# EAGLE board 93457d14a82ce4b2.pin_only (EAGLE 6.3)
REV: D

Size 66.04 x 50.8 mm. Coordinates in mm from the lower left corner, seen from the top.
Outline: 0,45.72 0,5.08 arc90 5.08,0 60.96,0 arc90 66.04,5.08 66.04,45.72 arc90 60.96,50.8 5.08,50.8 arc90 0,45.72
Copper layers (1*16): Top 0.035mm / dielectric 1.5mm / Bottom 0.035mm
Design rules "adafruit": minimum track width 8mil, minimum drill 15.5mil, track to track 8mil, track to pad 8mil, pad to pad 8mil, via to via 8mil, smd to smd 8mil, copper to edge 10mil, drill to drill 8mil, minimum pad ring 10mil, minimum via ring 8mil, stop-mask expansion 2mil, vias tented up to drill 20mil, thermal gap 10mil
tRestrict: area 24.7,24.1 to 24.8,24.4; area 7,19.9 to 7.5,20; area 22.1,34.8 to 22.9,36.2; area 22.2,32.8 to 22.9,34.2; area 22.2,31.8 to 22.7,32.3; area 22.2,30.2 to 22.9,31.1; area 22.4,27.3 to 22.7,29.7; area 23.2,25.3 to 24.3,25.9; area 25.3,25.3 to 31.1,25.8; area 49.5,9.7 to 49.9,9.8; 1 lines

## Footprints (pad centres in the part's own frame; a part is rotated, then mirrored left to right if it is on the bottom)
0805-NO = smd 1.3 x 1.5: 1 -0.95,0; 2 0.95,0
_0805MP = smd 1.2 x 1.3: 1 -1.016,0; 2 1.016,0
PANASONIC_C = smd 2.6 x 1.4: + 2.05,0; - -2.05,0
SOD-123 = smd 1.4 x 1.4: A 1.85,0; C -1.85,0
SMADIODE = smd 2.54 x 2.54: A 2.349,0; C -2.349,0
SOD-323 = smd 1.35 x 0.8: A 1.27,0; C -1.27,0
FIDUCIAL_1MM = smd 1 x 1: 1 0,0
TSSOP20-5.3MMBODY = smd 0.305 x 1.27: 1 -2.925,-3.618; 2 -2.275,-3.618; 3 -1.625,-3.618; 4 -0.975,-3.618; 5 -0.325,-3.618; 6 0.325,-3.618; 7 0.975,-3.618; 8 1.625,-3.618; 9 2.275,-3.618; 10 2.925,-3.618; 11 2.925,3.618; 12 2.275,3.618; 13 1.625,3.618; 14 0.975,3.618; 15 0.325,3.618; 16 -0.325,3.618; 17 -0.975,3.618; 18 -1.625,3.618; 19 -2.275,3.618; 20 -2.925,3.618
1X02_ROUND = drill 1 pad 1.778: 1 -1.27,0; 2 1.27,0
1X04_ROUND_76 = drill 1 pad 1.93: 1 -3.81,0; 2 -1.27,0; 3 1.27,0; 4 3.81,0
INDUCTOR_5X5MM_NR5040_NOTHERMALS = smd 1.8 x 4: P$1 -1.8,0; P$2 1.8,0
CHIPLED_0805_NOOUTLINE = smd 1.2 x 1.2: A 0,-1.05; C 0,1.05
SOT23-R = smd 0.635 x 1.016: 1 -0.95,-1; 2 0.95,-1; 3 0,1
RESPACK_4X0603 = smd 0.45 x 0.9: 1 -1.3,-0.85; 2 -0.4,-0.85; 3 0.4,-0.85; 4 1.3,-0.85; 5 1.3,0.85; 6 0.4,0.85; 7 -0.4,0.85; 8 -1.3,0.85
SOLDERJUMPER_ARROW_NOPASTE = smd 0.762 x 1.524: 1 -1.016,0; 2 1.016,0
SOLDERJUMPER_CLOSEDWIRE = smd 1.168 x 1.6: 1 -0.762,0; 2 0.762,0 | smd 0.635 x 0.203: WIRE 0,0
S-PQFP-G100 = smd 0.27 x 1.5: 1 -6,-7.75; 2 -5.5,-7.75; 3 -5,-7.75; 4 -4.5,-7.75; 5 -4,-7.75; 6 -3.5,-7.75; 7 -3,-7.75; 8 -2.5,-7.75; 9 -2,-7.75; 10 -1.5,-7.75; 11 -1,-7.75; 12 -0.5,-7.75; 13 0,-7.75; 14 0.5,-7.75; 15 1,-7.75; 16 1.5,-7.75; 17 2,-7.75; 18 2.5,-7.75; 19 3,-7.75; 20 3.5,-7.75; 21 4,-7.75; 22 4.5,-7.75; 23 5,-7.75; 24 5.5,-7.75; 25 6,-7.75; 51 6,7.75; 52 5.5,7.75; 53 5,7.75; 54 4.5,7.75; 55 4,7.75; 56 3.5,7.75; 57 3,7.75; 58 2.5,7.75; 59 2,7.75; 60 1.5,7.75; 61 1,7.75; 62 0.5,7.75; 63 0,7.75; 64 -0.5,7.75; 65 -1,7.75; 66 -1.5,7.75; 67 -2,7.75; 68 -2.5,7.75; 69 -3,7.75; 70 -3.5,7.75; 71 -4,7.75; 72 -4.5,7.75; 73 -5,7.75; 74 -5.5,7.75; 75 -6,7.75 | smd 1.5 x 0.27: 26 7.75,-6; 27 7.75,-5.5; 28 7.75,-5; 29 7.75,-4.5; 30 7.75,-4; 31 7.75,-3.5; 32 7.75,-3; 33 7.75,-2.5; 34 7.75,-2; 35 7.75,-1.5; 36 7.75,-1; 37 7.75,-0.5; 38 7.75,0; 39 7.75,0.5; 40 7.75,1; 41 7.75,1.5; 42 7.75,2; 43 7.75,2.5; 44 7.75,3; 45 7.75,3.5; 46 7.75,4; 47 7.75,4.5; 48 7.75,5; 49 7.75,5.5; 50 7.75,6; 76 -7.75,6; 77 -7.75,5.5; 78 -7.75,5; 79 -7.75,4.5; 80 -7.75,4; 81 -7.75,3.5; 82 -7.75,3; 83 -7.75,2.5; 84 -7.75,2; 85 -7.75,1.5; 86 -7.75,1; 87 -7.75,0.5; 88 -7.75,0; 89 -7.75,-0.5; 90 -7.75,-1; 91 -7.75,-1.5; 92 -7.75,-2; 93 -7.75,-2.5; 94 -7.75,-3; 95 -7.75,-3.5; 96 -7.75,-4; 97 -7.75,-4.5; 98 -7.75,-5; 99 -7.75,-5.5; 100 -7.75,-6 | drill 0.4: P$1 -4,4; P$2 -2,4; P$3 0,4; P$4 2,4; P$5 4,4; P$6 4,2; P$7 4,0; P$8 4,-2; P$9 4,-4; P$10 2,-4; P$11 0,-4; P$12 -2,-4; P$13 -4,-4; P$14 -4,-2; P$15 -4,0; P$16 -4,2 | smd 12 x 12: THERMAL 0,0
SOT23-5 = smd 0.55 x 1.2: 1 -0.95,-1.3; 2 0,-1.3; 3 0.95,-1.3; 4 0.95,1.3; 5 -0.95,1.3
SOT223-R = smd 1.3 x 1.3: 1 -2.3,-3.05; 2 0,-3.05; 3 2.3,-3.05 | smd 3.6 x 1.3: 4 0,3.05
MOUNTINGHOLE_3.0_PLATED = drill 3 pad 6.452: P$1 0,0
HDMI_MOLEX_47151-0001_DIMLAYER = smd 0.25 x 2.6: 1 4.5,0; 2 4,0; 3 3.5,0; 4 3,0; 5 2.5,0; 6 2,0; 7 1.5,0; 8 1,0; 9 0.5,0; 10 0,0; 11 -0.5,0; 12 -1,0; 13 -1.5,0; 14 -2,0; 15 -2.5,0; 16 -3,0; 17 -3.5,0; 18 -4,0; 19 -4.5,0 | drill 0.9 pad 1.65 long: P$1 -7.25,-0.76; P$2 7.25,-0.76 | drill 0.9 pad 1.5 long: P$3 7.25,-6.72; P$4 -7.25,-6.72
4UCONN_20329 = smd 1 x 2: BASE@1 -0.75,-2; BASE@2 0.75,-2 | smd 0.4 x 1.35: D+ 0,0.775; D- -0.65,0.775; GND 1.3,0.775; ID 0.65,0.775; VBUS -1.3,0.775 | drill 0.7 offset: SPRT@1 -3.3,0.9; SPRT@2 3.3,0.9 | drill 0.6 pad 2.5 square: SPRT@3 -3.6,-1.9; SPRT@4 3.6,-1.9 | hole 0.7: -1.95,0; 1.95,0
4-1734839-0 = smd 0.25 x 1.1: 1 -9.75,-2.54; 2 -9.25,-2.54; 3 -8.75,-2.54; 4 -8.25,-2.54; 5 -7.75,-2.54; 6 -7.25,-2.54; 7 -6.75,-2.54; 8 -6.25,-2.54; 9 -5.75,-2.54; 10 -5.25,-2.54; 11 -4.75,-2.54; 12 -4.25,-2.54; 13 -3.75,-2.54; 14 -3.25,-2.54; 15 -2.75,-2.54; 16 -2.25,-2.54; 17 -1.75,-2.54; 18 -1.25,-2.54; 19 -0.75,-2.54; 20 -0.25,-2.54; 21 0.25,-2.54; 22 0.75,-2.54; 23 1.25,-2.54; 24 1.75,-2.54; 25 2.25,-2.54; 26 2.75,-2.54; 27 3.25,-2.54; 28 3.75,-2.54; 29 4.25,-2.54; 30 4.75,-2.54; 31 5.25,-2.54; 32 5.75,-2.54; 33 6.25,-2.54; 34 6.75,-2.54; 35 7.25,-2.54; 36 7.75,-2.54; 37 8.25,-2.54; 38 8.75,-2.54; 39 9.25,-2.54; 40 9.75,-2.54 | smd 2.3 x 3.1: M1 11.4,-0.84; M2 -11.4,-0.84
RESONATOR-SMD = smd 0.7 x 1.7: 1 -1.2,0; 2 0,0; 3 1.2,0

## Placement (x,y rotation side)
C1  0.1uF  [0805-NO]  48.39,3.56 0 top
C2  0.1uF  [0805-NO]  26.3,20 270 top
C3  0.1uF  [0805-NO]  27.05,41.8 180 top
C4  0.1uF  [0805-NO]  43.56,3.3 0 top
C5  0.1uF  [0805-NO]  41.2,26.87 0 top
C6  0.1uF  [_0805MP]  40.8,35 90 top
C7  0.1uF  [0805-NO]  31.75,41.8 180 top
C8  0.1uF  [0805-NO]  20.25,40.25 0 top
C9  0.1uF  [0805-NO]  14.7,15.55 270 top
C10  0.1uF  [0805-NO]  20,20 270 top
C11  0.1uF  [0805-NO]  14.5,27.25 270 top
C12  10uF  [0805-NO]  12.42,14.41 270 top
C13  10uF  [0805-NO]  13.9,7.3 90 top
C14  10uF  [0805-NO]  22.9,7.3 90 top
C15  10uF  [0805-NO]  41.2,23.4 180 top
C16  10uF  [0805-NO]  37.52,45.33 270 top
C17  1uF  [0805-NO]  54,42.5 90 top
C18  1uF  [0805-NO]  51.8,42.5 90 top
C19  0.1uF  [0805-NO]  45,47.1 270 top
C20  0.1uF  [0805-NO]  24.3,42.9 270 top
C21  0.01uF  [0805-NO]  55.37,9.27 270 top
C22  0.01uF  [0805-NO]  59.31,10.29 180 top
C23  0.1uF  [0805-NO]  26.67,6.22 90 top
C24  0.01uF  [0805-NO]  53.98,12.7 270 top
C25  0.01uF  [0805-NO]  52.2,11.05 270 top
C26  100uF  [PANASONIC_C]  9.78,19.05 180 top
D1  MBR0540  [SOD-123]  47.3,40.2 180 top
D2  MM3Z24VT1G  [SMADIODE]  48.8,45.1 90 top
D3  2N4148  [SOD-323]  53.09,47.24 90 top
FB1  Ferrite  [_0805MP]  20.2,15.55 90 top
FB2  Ferrite  [_0805MP]  41.2,25.2 180 top
FB3  Ferrite  [_0805MP]  16.6,15.55 90 top
FB4  Ferrite  [_0805MP]  18.4,15.55 90 top
FB5  ferrite  [_0805MP]  57.66,12.06 0 top
FB6  ferrite  [_0805MP]  62.99,10.29 0 top
FB7  Ferrite  [_0805MP]  48.39,1.91 180 top
FB8  Ferrite  [_0805MP]  37.97,7.49 0 top
FB9  ferrite  [_0805MP]  56.52,16.38 0 top
FB10  ferrite  [_0805MP]  56.64,14.61 0 top
FID1  FIDUCIAL""  [FIDUCIAL_1MM]  37.19,41.95 0 top
FID2  FIDUCIAL""  [FIDUCIAL_1MM]  8.26,9.51 0 top
FID3  FIDUCIAL""  [FIDUCIAL_1MM]  45.88,14.76 0 top
IC1  AR1100_SSOP  [TSSOP20-5.3MMBODY]  46.1,7.75 90 top
JP1  [1X02_ROUND]  64.77,39.37 270 top
JP2  [1X02_ROUND]  2.92,21.34 0 top
JP6  [1X02_ROUND]  11.6,2.2 180 top
JP7  [1X04_ROUND_76]  13.97,48.26 0 top
L1  BRL3225T150K  [INDUCTOR_5X5MM_NR5040_NOTHERMALS]  41.5,41.4 0 top
LED1  Red  [CHIPLED_0805_NOOUTLINE]  54.48,2.04 270 top
LED2  Green  [CHIPLED_0805_NOOUTLINE]  23.98,3.56 270 top
LED3  Blue  [CHIPLED_0805_NOOUTLINE]  39.42,1.53 270 top
Q1  BSS138  [SOT23-R]  35.63,3.3 270 top
R1  10K  [0805-NO]  17.7,42.9 270 top
R2  10K  [0805-NO]  23.9,15.55 90 top
R3  10K  [0805-NO]  19.9,42.9 270 top
R4  10K  [0805-NO]  22.1,42.9 270 top
R5  10K  [_0805MP]  22,15.55 90 top
R6  33  [RESPACK_4X0603]  46.95,28.1 270 top
R7  33  [RESPACK_4X0603]  46.95,32.2 270 top
R8  33  [RESPACK_4X0603]  35.4,18.05 180 top
R9  33  [RESPACK_4X0603]  39.5,18.05 180 top
R10  33  [RESPACK_4X0603]  27.2,15.3 180 top
R11  33  [RESPACK_4X0603]  31.3,15.3 180 top
R12  33  [RESPACK_4X0603]  46.95,36.3 270 top
R13  10K  [_0805MP]  45.44,12.06 180 top
R14  1K  [0805-NO]  55.02,4.69 90 top
R15  3 ohm  [0805-NO]  31.75,47.03 270 top
R16  12 ohm  [0805-NO]  29.5,46.91 270 top
R17  12 ohm  [0805-NO]  26.99,47.03 270 top
R18  10K  [0805-NO]  35.3,47.1 90 top
R19  1K  [0805-NO]  24.8,6.23 90 top
R20  1K  [0805-NO]  39.42,3.43 180 top
R21  1K  [0805-NO]  30.94,6.73 0 top
SJ1  [SOLDERJUMPER_ARROW_NOPASTE]  19.63,15.75 270 bottom
SJ2  [SOLDERJUMPER_ARROW_NOPASTE]  22.1,15.75 90 bottom
SJ3  +50mA  [SOLDERJUMPER_ARROW_NOPASTE]  32.03,44.06 0 top
SJ4  +25mA  [SOLDERJUMPER_ARROW_NOPASTE]  26.95,44.02 0 top
SJ6  [SOLDERJUMPER_CLOSEDWIRE]  29.46,3.17 0 top
U1  TFP401  [S-PQFP-G100]  29,32 0 top
U2  24LC02BT-I/OT  [SOT23-5]  23.5,47.5 270 top
U3  LT1117(3V3)  [SOT223-R]  18.4,5.2 180 top
U4  FAN5333BSX  [SOT23-5]  41.4,47.5 90 top
U$31  MOUNTINGHOLE3.0  [MOUNTINGHOLE_3.0_PLATED]  5.08,45.72 0 top
U$32  MOUNTINGHOLE3.0  [MOUNTINGHOLE_3.0_PLATED]  60.96,45.72 0 top
U$33  MOUNTINGHOLE3.0  [MOUNTINGHOLE_3.0_PLATED]  60.96,5.08 0 top
U$34  MOUNTINGHOLE3.0  [MOUNTINGHOLE_3.0_PLATED]  5.08,5.08 0 top
U$80  [PCBFEAT-REV-056]  34.54,7.37 0 top
U$81  [ADAFRUIT_TEXT_20MM]  53.85,16.26 90 top
X1  47151-0001  [HDMI_MOLEX_47151-0001_DIMLAYER]  9.25,32 270 top
X2  microUSB  [4UCONN_20329]  4.38,14.5 270 top
X3  XF2-40-RARBT  [4-1734839-0]  62.2,24.55 270 top
Y1  12MHz  [RESONATOR-SMD]  51.99,4.92 90 top

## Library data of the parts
C1 C4 C12-C23 C26 D1-D3 FB1-FB8 IC1 JP1 JP6 JP7 L1 LED1-LED3 Q1 R1 R6-R21 SJ6 U1-U4 U$80 U$81 X1 X2 = microbuilder
C2 C3 C5-C11 R2-R5 = microbuilder; COMPANY: ADAFRUIT INDUSTRIES; DRAWN: KTOWN; REV: A
C24 C25 FB9 FB10 JP2 = microbuilder; COMPANY: ADAFRUIT INDUSTRIES; DRAWN: FZHAO; REV: C
FID1-FID3 SJ1 SJ3 SJ4 U$31-U$34 = microbuilder; BOM: EXCLUDE
SJ2 = microbuilder; BOM: EXCLUDE; COMPANY: ADAFRUIT INDUSTRIES; DRAWN: KTOWN; REV: A
X3 = adafruit
Y1 = SparkFun

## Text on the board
tPlace: +5V | GND | SCL | SDA | EDID / EEPROM | GND | Backlight | TFP401 | 5V | GND | 40-Pin TTL RGB | HDMI/DVI Decoder Breakout | (w/AR1100 USB Touch) | GND | +3V3 | PWR | HDMI | Touch
bPlace: +5V | GND | SCL | SDA | Backlite / Jumpers | +25mA | +100mA | GND | Backlight | 5V | GND | OCK_INV | ST | GND | +3V3

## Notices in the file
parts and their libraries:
microbuilder: This work is placed in the public domain, and may be freely used for commercial and non-commercial work with the following conditions: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
SparkFun: Licensing: CC v3.0 Share-Alike You are welcome to use this library for commercial purposes.
